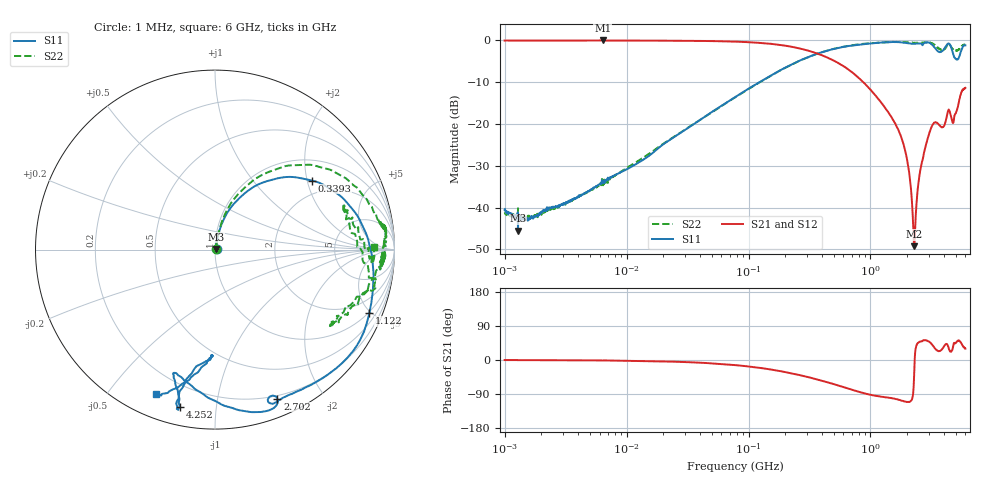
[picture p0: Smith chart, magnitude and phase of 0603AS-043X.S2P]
!s-Parameter Generated by FASTRON Sdn. Bhd.
!FASTRON P/N : 0603AS-043X
!Keysight Technologies: E5071C_MY46733604_B.14.02
!Date: Thu Nov 23 11:12:33 2023
!Version  :Rev01  Thu Nov 23 11:12:33 2023
!Data & Calibration Information:
!Freq  S11:SOLT2(ON)  S21:SOLT2(ON)  S12:SOLT2(ON)  S22:SOLT2(ON)
!PortZ  Port1:50+j0  Port2:50+j0
!When reading reference impedance value at option line is always used.
! Remarks : This data is being provided solely for informational purposes.
# Hz S dB R 50
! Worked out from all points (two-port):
!   1601 points, 1 MHz to 6 GHz, reference 50 ohm
!   highest |S21| = -0.04 dB at 6.378 MHz (marker M1); lowest = -49.2 dB at 2.279 GHz (marker M2)
!   |S21| within 3 dB of the highest: start of sweep to 354.7 MHz
!   lowest |S11| = -45.6 dB at 1.288 MHz (marker M3), VSWR 1.01, Z = 50.4 + j0.283 ohm
!   |S11| at or under -10 dB: start of sweep to 123.4 MHz
!   |S22| runs from -43.5 to -0.4 dB; largest |S21 - S12| = 0.0081
!   S11 on the Smith chart (normalised r, x): 1 MHz: 1.02, +0.01; 339.3 MHz: 1.56, +2.15; 1.122 GHz: 0.94, -4.90; 2.702 GHz: 0.17, -1.49; 4.252 GHz: 0.09, -0.80; 6 GHz: 0.10, -0.67
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1000000  -40.53 25.0  -0.06 -0.2  -0.07 -0.2  -41.14 25.5
1287650  -45.55 32.1  -0.07 -0.2  -0.05 -0.2  -40.18 19.4
4277066  -37.00 63.6  -0.07 -0.8  -0.07 -0.8  -37.12 63.5
6378092  -33.92 72.6  -0.04 -1.2  -0.08 -1.3  -35.11 73.4
1.823719e7  -25.80 78.3  -0.09 -3.3  -0.10 -3.3  -25.55 77.4
7.757876e7  -13.60 72.0  -0.31 -13.4  -0.32 -13.4  -13.65 74.1
1.643409e8  -7.88 58.9  -0.95 -26.9  -0.95 -26.8  -7.92 63.2
3.307917e8  -3.67 36.3  -2.74 -47.7  -2.73 -47.7  -3.70 46.1
3.392739e8  -3.55 35.3  -2.84 -48.6  -2.84 -48.6  -3.57 45.2
6.317636e8  -1.46 6.4  -6.61 -73.8  -6.61 -73.8  -1.41 25.1
1.121889e9  -0.63 -22.3  -13.55 -95.0  -13.57 -95.0  -0.59 8.6
1.414819e9  -0.43 -31.3  -17.46 -99.9  -17.48 -99.9  -0.42 6.8
1.928676e9  -0.61 -51.1  -26.55 -109.6  -26.55 -109.4  -0.42 3.4
2.077493e9  -0.75 -57.7  -31.73 -110.9  -31.75 -110.8  -0.57 -1.3
2.226311e9  -0.83 -62.9  -42.64 -93.3  -42.67 -93.2  -0.57 -1.8
2.27946e9  -0.83 -64.3  -49.24 -40.0  -49.32 -39.9  -0.61 -4.9
2.702095e9  -0.92 -67.3  -27.99 52.0  -27.96 52.1  -0.49 -3.0
3.17898e9  -0.95 -82.6  -20.67 41.8  -20.64 41.6  -0.63 -6.4
3.766207e9  -2.81 -108.4  -20.63 25.3  -20.64 25.1  -2.12 -32.1
4.252188e9  -0.95 -102.7  -17.71 41.6  -17.74 41.5  -1.09 -14.9
5.048685e9  -4.55 -91.1  -17.10 46.9  -17.12 46.9  -2.44 18.9
6e9  -1.21 -112.3  -11.40 30.0  -11.40 30.0  -1.04 0.8
